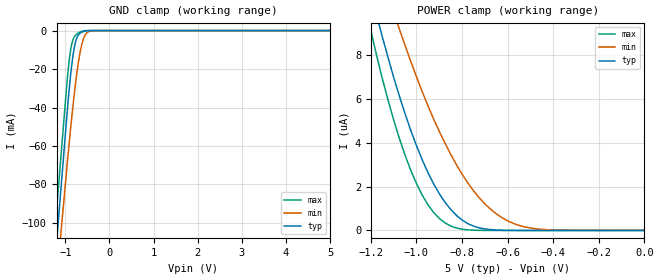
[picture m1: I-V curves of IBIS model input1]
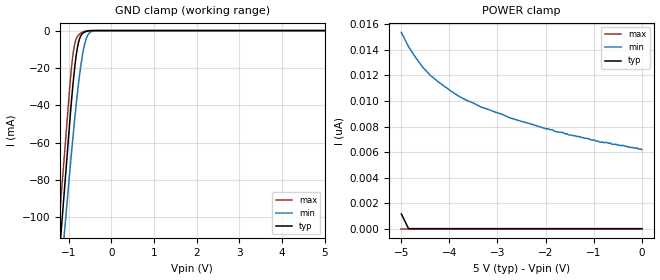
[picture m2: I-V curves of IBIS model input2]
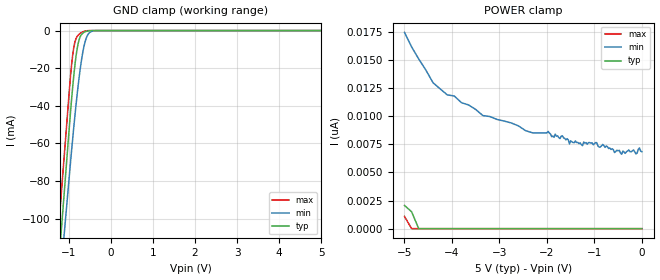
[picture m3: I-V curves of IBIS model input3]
|   Microchip Technology Inc.
|   93LC86C - 16 Kbit Microwire serial EEPROM
|   (Vcc = +2.5V to +5.5V)
|   150K Process
|   Copyright (C) 2018 Microchip Technology Inc.
[IBIS ver]   3.2
[File name]   93lc86c-e_st-5v.ibs
[File Rev]   1.0
[Date]   May 18, 2018
[Source]   Waveforms generated by SPICE simulation at Microchip.
   All other data taken from lab measurements at Microchip.
[Notes]   This IBIS model is for the Microchip 93LC86C device, a
   16 Kbit Microwire bus serial EEPROM manufactured on
   Microchip's 150K process, for automotive temp in
   a 4.4 mm, 8-lead TSSOP package operating at 5V.
[Disclaimer] Unauthorized reproduction and/or distribution is
   strictly restricted. All rights reserved.
   This information is provided to you for your convenience
   and use with Microchip products only. Microchip
   disclaims all liability arising from this information
   and its use.
   THIS INFORMATION IS PROVIDED "AS IS." MICROCHIP MAKES NO
   REPRESENTATION OR WARRANTIES OF ANY KIND WHETHER EXPRESS
   OR IMPLIED, WRITTEN OR ORAL, STATUTORY OR OTHERWISE,
   RELATED TO THE INFORMATION PROVIDED TO YOU, INCLUDING
   BUT NOT LIMITED TO ITS CONDITION, QUALITY, PERFORMANCE,
   MERCHANTABILITY, NON-INFRINGEMENT, OR FITNESS FOR
   PURPOSE. MICROCHIP IS NOT LIABLE, UNDER ANY
   CIRCUMSTANCES, FOR SPECIAL, INCIDENTAL OR CONSEQUENTIAL
   DAMAGES, FOR ANY REASON WHATSOEVER.
   It is your responsibility to ensure that your
   application meets with your specifications.
|   Component 93LC86C-E/ST
[Component]   93LC86C-E/ST
[Manufacturer]   Microchip Technology Inc.
[Package]
| variable   typ   min   max
R_pkg   99.09m   85.92m   112.26m
L_pkg   2.16nH   1.55nH   2.76nH
C_pkg   0.49pF   0.43pF   0.55pF
[Pin]  signal_name   model_name
1   CS   input1
2   CLK   input2
3   DI   input3
4   DO   driver
5   VSS   GND
6   ORG   input4
7   PE   input5
8   VCC   POWER
| Models and submodels in the file (6): input1 (Input), input2 (Input), input3 (Input), driver (3-state), input4 (Input), input5 (Input)
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|   Model input1
[Model]   input1
Model_type   Input
Vinl = 0.8
Vinh = 2.0
C_comp   5.00pF   5.00pF   5.00pF
[Temperature Range]   25.00   125.00   -40.00
[Voltage Range]   5.00V   2.50V   5.50V
[Pullup Reference]   5.00V   5.00V   5.00V
[POWER Clamp Reference]   5.00V   5.00V   5.00V
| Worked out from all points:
|   GND clamp passes 1 mA (typ) near -0.64 V on its own axis
[GND_clamp]
| voltage   I(typ)   I(min)   I(max)
-5V       -1.185A    -1.088A    -1.164A
-1.25V    -124.7mA   -142.9mA   -107.7mA
-1.1V     -82.25mA   -105.1mA   -65.49mA
-975mV    -46.9mA    -73.63mA   -30.29mA
-900mV    -27.63mA   -55.45mA   -13.24mA
-850mV    -17.05mA   -44.02mA   -6.528mA
-775mV    -6.431mA   -28.57mA   -2.594mA
-725mV    -3.025mA   -19.72mA   -1.545mA
-650mV    -1.099mA   -9.514mA   -587.6uA
-550mV    -229.9uA   -2.316mA   -60.37uA
-375mV    -1.003uA   -77.3uA    -34.54nA
5V        10pA       4.131nA    10pA
[POWER_clamp]
| voltage   I(typ)   I(min)   I(max)
-5V       24.92uA    17.87uA    30.57uA
-1.2V     10.85uA    13.73uA    9.102uA
-1.15V    8.826uA    11.48uA    6.925uA
-1.075V   6.121uA    9.171uA    4.192uA
-1.025V   4.559uA    7.7uA      2.738uA
-975mV    3.221uA    6.33uA     1.613uA
-900mV    1.679uA    4.516uA    551.6nA
-800mV    477.7nA    2.57uA     57.52nA
-675mV    39nA       971.2nA    1.073nA
-600mV    5.799nA    438nA      10pA
-500mV    10pA       112.8nA    10pA
0V        10pA       5.633nA    10pA
|   Model input2
[Model]   input2
Model_type   Input
Vinl = 0.8
Vinh = 2.0
C_comp   5.00pF   5.00pF   5.00pF
[Temperature Range]   25.00   125.00   -40.00
[Voltage Range]   5.00V   2.50V   5.50V
[Pullup Reference]   5.00V   5.00V   5.00V
[POWER Clamp Reference]   5.00V   5.00V   5.00V
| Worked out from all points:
|   GND clamp passes 1 mA (typ) near -0.64 V on its own axis
[GND_clamp]
| voltage   I(typ)   I(min)   I(max)
-5V       -1.223A    -1.118A    -1.194A
-1.25V    -129.2mA   -147.1mA   -110mA
-1.1V     -85.41mA   -108.3mA   -66.57mA
-950mV    -41.88mA   -69.47mA   -23.72mA
-900mV    -29.05mA   -57.22mA   -13.01mA
-850mV    -18.04mA   -45.46mA   -6.327mA
-800mV    -9.75mA    -34.56mA   -3.315mA
-750mV    -4.639mA   -24.77mA   -1.974mA
-675mV    -1.564mA   -12.9mA    -827uA
-550mV    -237.5uA   -2.356mA   -55.38uA
-375mV    -1.103uA   -75.11uA   -28.42nA
5V        10pA       4.594nA    10pA
[POWER_clamp]
| voltage   I(typ)   I(min)   I(max)
-5V       1.163nA    15.36nA    10pA
-4.85V    10pA       14.24nA    10pA
-4.55V    10pA       12.62nA    10pA
-4.4V     10pA       12.01nA    10pA
-3.95V    10pA       10.73nA    10pA
-3.65V    10pA       10.06nA    10pA
-3.35V    10pA       9.533nA    10pA
-2.75V    10pA       8.688nA    10pA
-1.975V   10pA       7.796nA    10pA
-875mV    10pA       6.786nA    10pA
-400mV    10pA       6.538nA    10pA
0V        10pA       6.189nA    10pA
|   Model input3
[Model]   input3
Model_type   Input
Vinl = 0.8
Vinh = 2.0
C_comp   5.00pF   5.00pF   5.00pF
[Temperature Range]   25.00   125.00   -40.00
[Voltage Range]   5.00V   2.50V   5.50V
[Pullup Reference]   5.00V   5.00V   5.00V
[POWER Clamp Reference]   5.00V   5.00V   5.00V
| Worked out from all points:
|   GND clamp passes 1 mA (typ) near -0.64 V on its own axis
[GND_clamp]
| voltage   I(typ)   I(min)   I(max)
-5V       -1.21A     -1.101A    -1.186A
-1.25V    -128.6mA   -145.5mA   -108.9mA
-1.1V     -85.37mA   -107.3mA   -65.78mA
-950mV    -42.29mA   -69.1mA    -23.23mA
-900mV    -29.54mA   -57.04mA   -12.65mA
-850mV    -18.52mA   -45.46mA   -6.148mA
-800mV    -10.12mA   -34.69mA   -3.259mA
-750mV    -4.849mA   -25mA      -1.953mA
-675mV    -1.617mA   -13.17mA   -815.9uA
-550mV    -248.8uA   -2.46mA    -53.39uA
-375mV    -1.248uA   -80.38uA   -26.23nA
5V        10pA       5.036nA    10pA
[POWER_clamp]
| voltage   I(typ)   I(min)   I(max)
-5V       2.074nA    17.43nA    1.096nA
-4.85V    1.507nA    16.14nA    10pA
-4.7V     10pA       15.07nA    10pA
-4.4V     10pA       12.97nA    10pA
-3.35V    10pA       10.05nA    10pA
-2.3V     10pA       8.512nA    10pA
-1.675V   10pA       8.255nA    10pA
-1.525V   10pA       7.532nA    10pA
-950mV    10pA       7.642nA    10pA
-425mV    10pA       6.614nA    10pA
-50mV     10pA       7.17nA     10pA
0V        10pA       6.834nA    10pA
